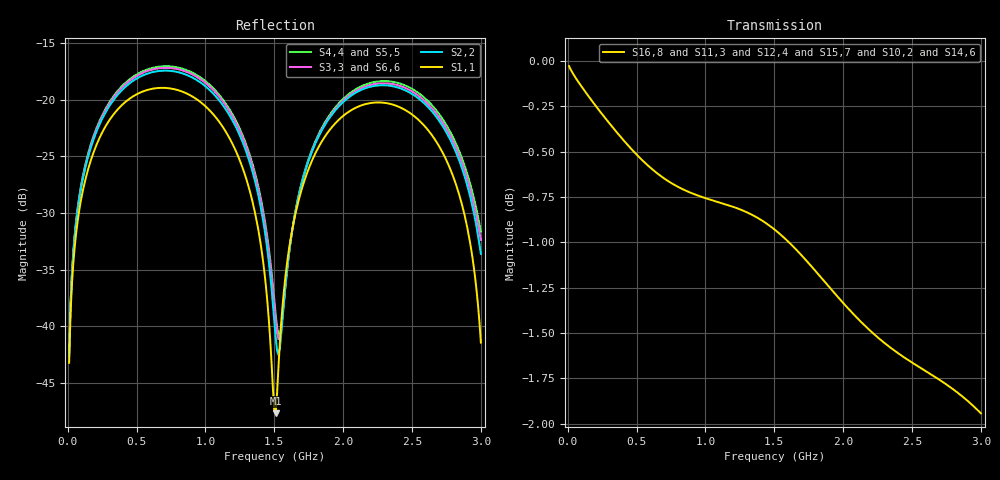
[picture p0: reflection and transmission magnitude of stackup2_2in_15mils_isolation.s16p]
! Touchstone file from project
# GHZ S RI R 50.000000
! Modal data exported
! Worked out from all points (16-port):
!   300 points, 10 MHz to 3 GHz, reference 50 ohm
!   strongest paths, dB at 10 MHz, 760 MHz, 1.51 GHz, 2.26 GHz, 3 GHz:
!     S16,8: 0.0, -0.7, -0.9, -1.5, -1.9
!     S11,3: 0.0, -0.7, -0.9, -1.6, -2.0
!     S12,4: 0.0, -0.7, -0.9, -1.6, -2.0
!     S15,7: 0.0, -0.7, -0.9, -1.6, -2.0
!     S10,2: 0.0, -0.7, -0.9, -1.6, -2.0
!     S14,6: 0.0, -0.7, -0.9, -1.6, -2.0
!   lowest |S11| = -47.7 dB at 1.51 GHz (marker M1), VSWR 1.01, Z = 50.4 + j0.0652 ohm
!   |S11| at or under -10 dB: start of sweep to end of sweep
